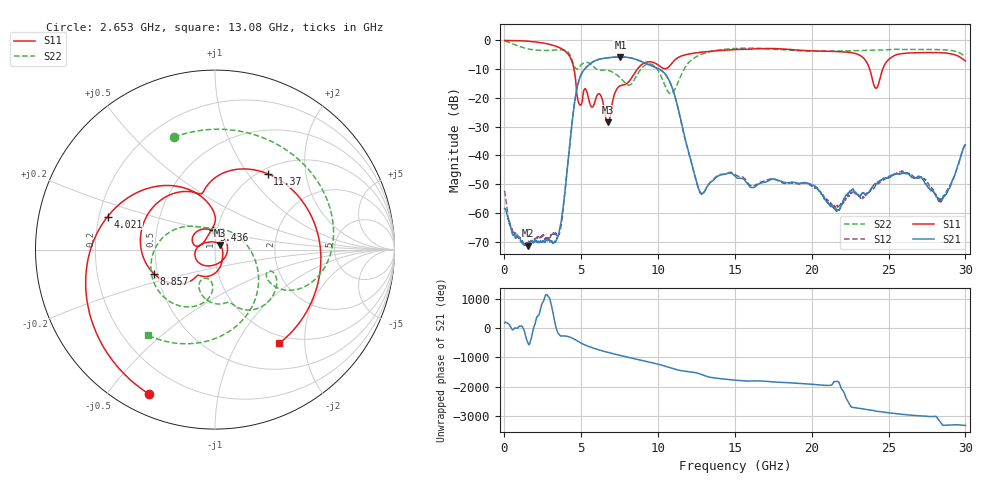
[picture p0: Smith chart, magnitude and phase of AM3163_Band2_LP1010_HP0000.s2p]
!Agilent Technologies,E8364B,MY43040894,A.07.50.67
!Agilent E8364B: A.07.50.67
!Date: Thursday, August 20, 2020 12:03:59
!Correction: S11(Full 2 Port(1,2))
!S21(Full 2 Port(1,2))
!S12(Full 2 Port(1,2))
!S22(Full 2 Port(1,2))
!S2P File: Measurements: S11, S21, S12, S22:
# Hz S  dB  R 50
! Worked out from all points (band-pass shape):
!   3201 points, 10 MHz to 30 GHz, reference 50 ohm
!   highest |S21| = -5.76 dB at 7.545 GHz (marker M1); lowest = -71.4 dB at 1.5 GHz (marker M2)
!   |S21| within 3 dB of the highest: 5.448 GHz to 9.548 GHz (4.1 GHz wide, 54.7 % of centre)
!   lowest |S11| = -28.5 dB at 6.73 GHz (marker M3), VSWR 1.08, Z = 52.8 + j2.69 ohm
!   |S11| at or under -10 dB: 4.528 GHz to 8.646 GHz (4.118 GHz wide, 62.5 % of centre); 23.77 GHz to 24.62 GHz (849.3 MHz wide, 3.51 % of centre)
!   |S22| runs from -18.5 to -0.2 dB; largest |S21 - S12| = 0.0043
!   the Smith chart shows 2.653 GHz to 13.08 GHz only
!   S11 on the Smith chart (normalised r, x): 2.653 GHz: 0.09, -0.64; 4.021 GHz: 0.23, +0.14; 5.436 GHz: 0.96, +0.21; 8.857 GHz: 0.48, -0.15; 11.37 GHz: 1.08, +1.25; 13.08 GHz: 0.87, -1.53
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1e7  -0.03 -2.8  -58.45 173.7  -52.29 -54.1  -0.23 -9.1
6.84775e8  -0.06 -28.2  -67.97 4.1  -67.14 78.9  -1.54 -83.1
1.500128e9  -0.27 -62.6  -71.42 -108.6  -71.05 -76.7  -2.92 -161.2
2.652869e9  -1.06 -114.4  -69.98 14.0  -69.34 -171.7  -3.52 110.0
3.561941e9  -2.49 -163.6  -66.64 145.3  -67.34 -45.0  -3.28 43.9
4.021162e9  -4.07 162.9  -48.40 85.6  -47.97 83.9  -3.59 5.2
5.014581e9  -22.12 157.1  -11.63 -160.3  -11.63 -160.5  -8.40 -25.6
5.436316e9  -19.37 94.7  -8.81 102.5  -8.84 102.2  -7.72 -50.2
6.045488e9  -18.95 -134.1  -6.74 -7.5  -6.77 -7.6  -10.16 -73.3
6.729634e9  -28.46 42.4  -6.03 -108.7  -6.06 -108.8  -10.43 -90.1
7.544988e9  -15.77 -113.5  -5.76 145.8  -5.78 145.8  -13.04 -113.7
8.85705e9  -8.75 -158.2  -7.22 -14.1  -7.21 -14.3  -10.11 -104.3
1.000979e10  -8.57 120.1  -9.81 -153.1  -9.86 -153.2  -10.58 166.3
1.136871e10  -5.77 55.2  -25.12 1.8  -25.27 1.2  -13.67 -5.5
1.308377e10  -3.96 -55.6  -51.86 164.7  -51.97 166.7  -4.36 -127.8
1.5005e10  -3.19 -140.0  -47.19 20.6  -46.58 22.6  -2.82 156.2
1.777908e10  -2.89 95.9  -48.63 -44.5  -48.73 -48.1  -3.15 46.5
2.000958e10  -3.65 -17.8  -50.25 -117.8  -50.61 -117.6  -3.74 -38.2
2.295235e10  -4.77 -139.3  -53.37 152.2  -53.82 148.1  -3.57 -125.4
2.500479e10  -6.65 -132.6  -47.82 -9.0  -47.29 -4.2  -3.26 -176.3
2.837867e10  -4.29 106.3  -55.23 27.1  -55.96 -89.3  -3.23 95.2
3e10  -7.11 44.6  -36.39 -81.7  -35.95 -79.7  -5.54 46.8
